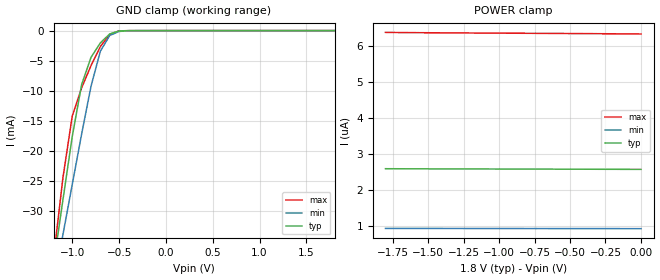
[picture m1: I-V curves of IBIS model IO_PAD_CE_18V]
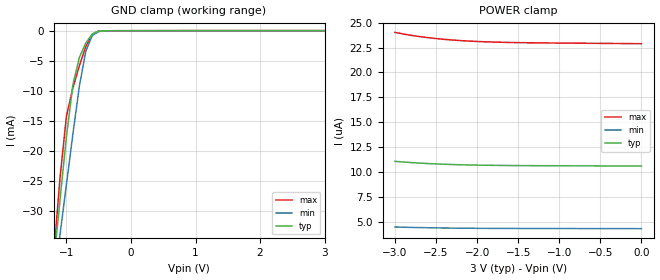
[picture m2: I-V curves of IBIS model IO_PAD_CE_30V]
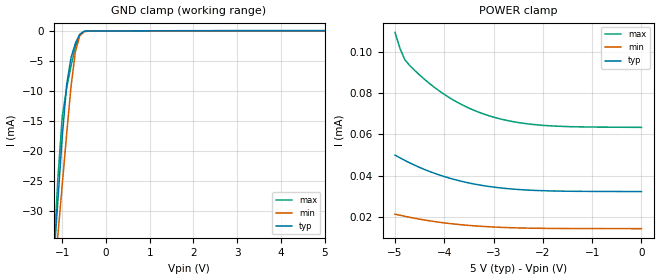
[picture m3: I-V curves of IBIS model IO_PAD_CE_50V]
[IBIS Ver]   3.2
[Comment Char]   |_char
[File name]   ra4000_4w.ibs
[File Rev]   1.0
[Date]   2021/11/25 18:33:27
[Source]
[Notes]
[Disclaimer]
This information is for modeling purposes only, and is not guaranteed.
Property of SEIKO EPSON Corp.,
unauthorized reproduction and/or distribution is strictly prohibited.
[Copyright]
Copyright 2021, SEIKO EPSON Corp.
[Component]   ra4000_4w
Si_location Pin
Timing_location Pin
[Manufacturer]   SEIKO EPSON Corp.
| PKG
[Package]
R_pkg   267m   NA   NA
L_pkg   2.8nH   NA   NA
C_pkg   0.70pF   NA   NA
[Pin] signal_name   model_name
1   DI   IO_PAD_DI_select
2   VDD   POWER
3   CE   IO_PAD_CE_select
4   /INT   IO_PAD_XINT_select
5   /RST   IO_PAD_XRST_select
6   EVIN2   IO_PAD_EVIN_select
7   DO   IO_PAD_DO_select
8   CLK   IO_PAD_CLK_select
9   GND   GND
10   SOUT   IO_PAD_SOUT_select
[Model Selector]  IO_PAD_CE_select
IO_PAD_CE_18V  18V mode
IO_PAD_CE_30V  30V mode
IO_PAD_CE_50V  50V mode
[Model Selector]  IO_PAD_CLK_select
IO_PAD_CLK_18V  18V mode
IO_PAD_CLK_30V  30V mode
IO_PAD_CLK_50V  50V mode
[Model Selector]  IO_PAD_DI_select
IO_PAD_DI_18V  18V mode
IO_PAD_DI_30V  30V mode
IO_PAD_DI_50V  50V mode
[Model Selector]  IO_PAD_DO_select
IO_PAD_DO_18V  18V mode
IO_PAD_DO_30V  30V mode
IO_PAD_DO_50V  50V mode
[Model Selector]  IO_PAD_EVIN_select
IO_PAD_EVIN_18V  18V mode
IO_PAD_EVIN_30V  30V mode
IO_PAD_EVIN_50V  50V mode
[Model Selector]  IO_PAD_SOUT_select
IO_PAD_SOUT_18V  18V mode
IO_PAD_SOUT_30V  30V mode
IO_PAD_SOUT_50V  50V mode
[Model Selector]  IO_PAD_XINT_select
IO_PAD_XINT_18V  18V mode
IO_PAD_XINT_30V  30V mode
IO_PAD_XINT_50V  50V mode
[Model Selector]  IO_PAD_XRST_select
IO_PAD_XRST_18V  18V mode
IO_PAD_XRST_30V  30V mode
IO_PAD_XRST_50V  50V mode
| Models and submodels in the file (24): IO_PAD_CE_18V (Input), IO_PAD_CE_30V (Input), IO_PAD_CE_50V (Input), IO_PAD_CLK_18V (Input), IO_PAD_CLK_30V (Input), IO_PAD_CLK_50V (Input), IO_PAD_DI_18V (Input), IO_PAD_DI_30V (Input), IO_PAD_DI_50V (Input), IO_PAD_DO_18V (3-state), IO_PAD_DO_30V (3-state), IO_PAD_DO_50V (3-state), IO_PAD_EVIN_18V (Input), IO_PAD_EVIN_30V (Input), IO_PAD_EVIN_50V (Input), IO_PAD_SOUT_18V (3-state), IO_PAD_SOUT_30V (3-state), IO_PAD_SOUT_50V (3-state), IO_PAD_XINT_18V (Open_drain), IO_PAD_XINT_30V (Open_drain), IO_PAD_XINT_50V (Open_drain), IO_PAD_XRST_18V (Open_drain), IO_PAD_XRST_30V (Open_drain), IO_PAD_XRST_50V (Open_drain)
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[Model]   IO_PAD_CE_18V
Model_type Input
Polarity Non-Inverting
Vinh=1.26
Vinl=0.54
C_comp   2.5p   2.0p   3.0p
[Temperature Range] 25   125   -40
[Voltage Range]   1.80   1.60   2.00
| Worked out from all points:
|   GND clamp passes 1 mA (typ) near -0.63 V on its own axis
[GND Clamp]
-1.8V     -104.1mA   -95.66mA   -119.4mA
-1.2V     -38.93mA   -42.42mA   -37.92mA
-1.1V     -28.21mA   -33.99mA   -24.54mA
-1V       -17.61mA   -25.59mA   -14.21mA
-900mV    -8.985mA   -17.22mA   -9.521mA
-800mV    -4.454mA   -9.272mA   -5.829mA
-700mV    -2.038mA   -3.423mA   -2.649mA
-600mV    -550.5uA   -805.9uA   -615.9uA
-500mV    -61.05uA   -137.3uA   -43.7uA
-400mV    -6.324uA   -18.27uA   -7.016uA
1.8V      2.562uA    917nA      6.314uA
[POWER Clamp]
-1.8V     2.58uA     923.3nA    6.365uA
-1.7V     2.579uA    922.8nA    6.361uA
-1.6V     2.577uA    922.3nA    6.358uA
-1.5V     2.576uA    921.9nA    6.355uA
-1.3V     2.574uA    921.2nA    6.35uA
-800mV    2.57uA     919.4nA    6.34uA
-500mV    2.567uA    918.3nA    6.334uA
-200mV    2.564uA    917nA      6.326uA
0V        2.562uA    916nA      6.32uA
[Model]   IO_PAD_CE_30V
Model_type Input
Polarity Non-Inverting
Vinh=2.10
Vinl=0.90
C_comp   2.5p   2.0p   3.0p
[Temperature Range] 25   125   -40
[Voltage Range]   3.00   2.70   3.30
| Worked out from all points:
|   GND clamp passes 1 mA (typ) near -0.63 V on its own axis
[GND Clamp]
-3V       -252.2mA   -212.5mA   -302.7mA
-1.2V     -38.93mA   -42.42mA   -37.92mA
-1.1V     -28.22mA   -33.99mA   -24.54mA
-1V       -17.62mA   -25.59mA   -14.21mA
-900mV    -8.991mA   -17.22mA   -9.528mA
-800mV    -4.458mA   -9.276mA   -5.835mA
-700mV    -2.042mA   -3.427mA   -2.655mA
-600mV    -553.6uA   -808uA     -621uA
-500mV    -63.69uA   -138.7uA   -48.01uA
-400mV    -8.461uA   -19.41uA   -10.52uA
3V        10.59uA    4.303uA    22.86uA
[POWER Clamp]
-3V       11.06uA    4.47uA     24.02uA
-2.9V     11uA       4.446uA    23.86uA
-2.8V     10.94uA    4.425uA    23.72uA
-2.7V     10.89uA    4.406uA    23.6uA
-2.6V     10.84uA    4.39uA     23.49uA
-2.5V     10.8uA     4.377uA    23.4uA
-2.3V     10.74uA    4.355uA    23.25uA
-2.2V     10.72uA    4.347uA    23.2uA
-2V       10.68uA    4.335uA    23.11uA
-1.7V     10.65uA    4.324uA    23.03uA
-1.4V     10.63uA    4.317uA    22.98uA
0V        10.59uA    4.298uA    22.88uA
[Model]   IO_PAD_CE_50V
Model_type Input
Polarity Non-Inverting
Vinh=3.50
Vinl=1.50
C_comp   2.5p   2.0p   3.0p
[Temperature Range] 25   125   -40
[Voltage Range]   5.00   4.50   5.50
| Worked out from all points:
|   GND clamp passes 1 mA (typ) near -0.63 V on its own axis
[GND Clamp]
-5V       -507.1mA   -412.9mA   -622.2mA
-1.2V     -38.93mA   -42.42mA   -37.92mA
-1.1V     -28.22mA   -34mA      -24.54mA
-1V       -17.62mA   -25.59mA   -14.22mA
-900mV    -8.995mA   -17.22mA   -9.533mA
-800mV    -4.462mA   -9.28mA    -5.841mA
-700mV    -2.045mA   -3.431mA   -2.66mA
-600mV    -556.8uA   -810.1uA   -625.1uA
-500mV    -66.4uA    -140.4uA   -51.53uA
-300mV    -5.693uA   -4.551uA   -9.437uA
5V        32.2uA     14.2uA     63.31uA
[POWER Clamp]
-5V       49.93uA    21.25uA    109.6uA
-4.9V     48.6uA     20.7uA     101.8uA
-4.8V     47.34uA    20.18uA    96.23uA
-4.6V     45.01uA    19.23uA    91.07uA
-4.3V     41.99uA    18uA       84.72uA
-4V       39.49uA    16.99uA    79.43uA
-3.7V     37.48uA    16.19uA    75.14uA
-3.3V     35.47uA    15.4uA     70.77uA
-2.7V     33.6uA     14.69uA    66.63uA
-2.1V     32.71uA    14.37uA    64.59uA
-1.4V     32.35uA    14.24uA    63.73uA
0V        32.2uA     14.18uA    63.4uA
